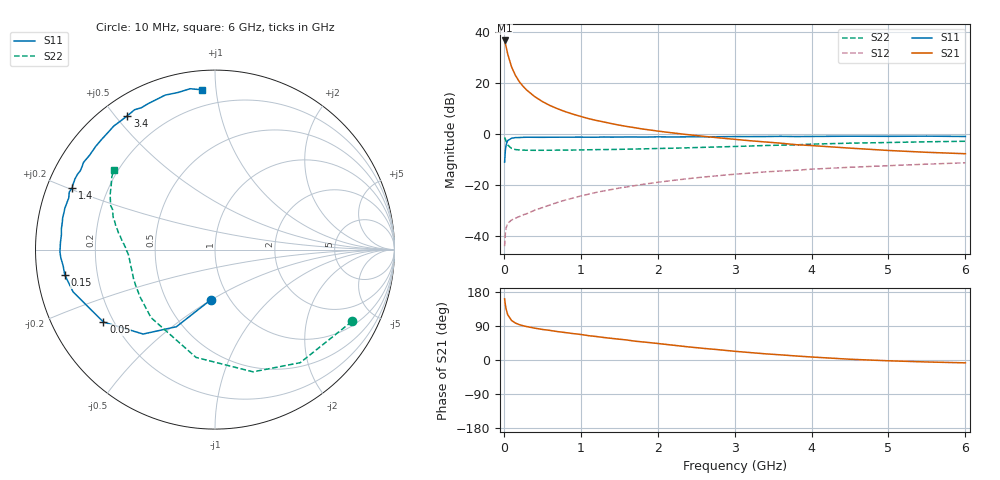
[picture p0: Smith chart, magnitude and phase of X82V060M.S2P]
! SIEMENS Small Signal Semiconductors
! BFP136W
! Si NPN RF Bipolar Junction Transistor in SOT343
! VCE = 2 V  IC = 60 mA
! Common Emitter S-Parameters:  September  1994
# GHz  S  MA  R  50
!  f  S11  S21  S12  S22
! GHz  MAG  ANG  MAG  ANG  MAG  ANG  MAG  ANG
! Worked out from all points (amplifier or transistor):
!   40 points, 10 MHz to 6 GHz, reference 50 ohm
!   highest |S21| = 36.8 dB at 10 MHz (marker M1)
!   |S21| within 3 dB of that: start of sweep to 33.35 MHz
!   unconditionally stable (mu >= 1): 538.8 MHz to 2.875 GHz
!   at 200 MHz: K = 0.61, MSG = 26.6 dB, |S12| = -32.5 dB
!   at 1.5 GHz: K = 1.11, MAG = 10.4 dB, |S12| = -21.3 dB
!   at 6 GHz: K = 0.97, MSG = 1.8 dB, |S12| = -11.3 dB
!   S11 on the Smith chart (normalised r, x): 10 MHz: 0.82, -0.50; 50 MHz: 0.16, -0.29; 150 MHz: 0.08, -0.08; 1.4 GHz: 0.07, +0.20; 3.4 GHz: 0.07, +0.54; 6 GHz: 0.10, +0.92
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0.01  0.2789 -94.4  69.29 161.5  0.0062 71.2  0.8613 -27.7
0.02  0.4806 -116.6  60.36 145.7  0.0111 58.3  0.7889 -53.0
0.03  0.6177 -130.4  51.77 134.1  0.0142 49.6  0.7133 -72.7
0.05  0.7411 -147.0  37.54 119.7  0.0174 38.6  0.6099 -100.0
0.1  0.8249 -163.4  20.97 104.4  0.0203 32.3  0.5203 -133.3
0.15  0.8488 -170.4  14.3 97.5  0.022 34.0  0.4937 -147.7
0.2  0.8508 -173.9  10.75 93.4  0.0237 36.7  0.4852 -155.5
0.25  0.86 -176.9  8.675 90.4  0.0256 39.6  0.4818 -160.5
0.3  0.8641 -179.1  7.25 88.1  0.0271 42.6  0.4786 -163.8
0.4  0.8619 177.2  5.459 84.1  0.0316 47.5  0.4775 -168.2
0.5  0.8597 174.6  4.354 80.7  0.0355 51.3  0.4783 -171.1
0.6  0.8636 172.4  3.632 78.1  0.0402 53.9  0.479 -173.0
0.7  0.8643 169.8  3.131 74.9  0.0452 56.0  0.4807 -174.3
0.9  0.8664 166.3  2.452 69.7  0.0549 58.3  0.4834 -176.8
1.1  0.8651 162.0  2.007 64.2  0.0653 59.2  0.4888 -178.4
1.4  0.8672 156.8  1.6 57.1  0.0809 59.5  0.4953 179.4
2.2  0.8744 143.1  1.048 39.1  0.122 55.1  0.5252 173.5
3.2  0.889 126.0  0.736 19.6  0.17 46.1  0.5792 164.5
3.4  0.8913 123.2  0.697 16.3  0.1798 44.1  0.5938 162.6
4.5  0.9044 107.9  0.527 2.0  0.2213 33.8  0.6598 152.3
5.5  0.907 98.8  0.436 -5.2  0.2548 25.9  0.7027 144.9
6  0.8929 94.5  0.409 -7.5  0.2715 21.4  0.719 141.7
